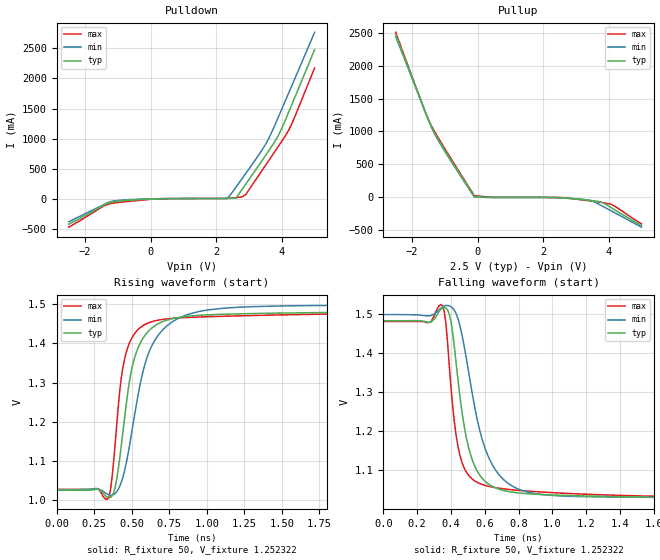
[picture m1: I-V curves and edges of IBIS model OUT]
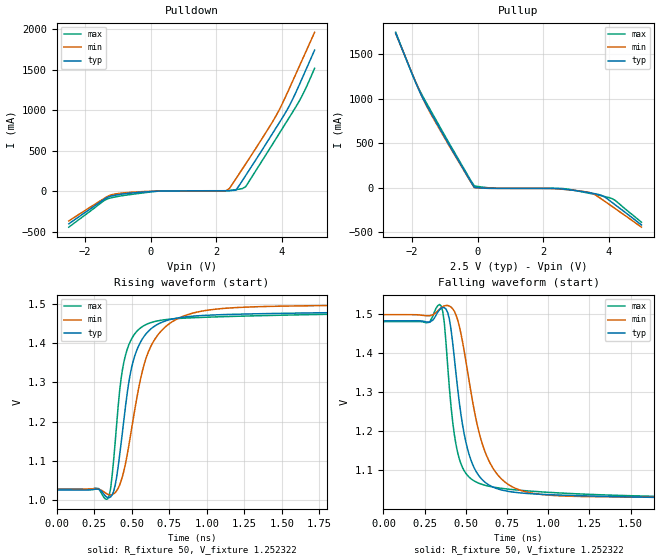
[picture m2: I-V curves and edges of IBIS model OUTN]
|   IBIS File of SG2520VHN D
|   LVDS, Vcc=2.5V, Io=4.5mA, fo<=212.5MHz
[IBIS Ver]   3.2
[File Name]   sg2520vhn_45m_25v.ibs
[File Rev]   1.0
[Date]   Sep. 16, 2020
[Source]
Fairchild Ensigna Lab's Method
[Notes]
Created by Minoru Kozaki
[Disclaimer]
Seiko Epson Corporation makes no warranty with respect to the
information contained herein.
[Copyright]
Copyright(C) 2020, Seiko Epson Corporation. All rights reserved.
|   Component
[Component]   SG2520VHN
[Manufacturer]  Seiko Epson Corporation
[Package]
R_pkg   17.7m   NA   NA
L_pkg   235p   NA   NA
C_pkg   208f   NA   NA
[Pin]   signal_name   model_name   R_pin   L_pin   C_pin
1   OE/ST   NC
2   NC   NC
3   GND   GND
4   OUT   OUT   17.7m   235p   208f
5   OUTN   OUTN   10.4m   129p   221f
6   VCC   POWER
[Diff Pin] inv_pin  vdiff  tdelay_typ
4   5   0   0
| Models and submodels in the file (2): OUT (Output), OUTN (Output)
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|   Model OUT
[Model]   OUT
Model_type   Output
Polarity   Non-Inverting
Vref = 1.25
Vmeas = 1.25
Rref = 50
Cref = 0
C_comp   4.5p   4.5p   4.5p
[Temperature Range]   25   105   -40
[Voltage Range]   2.5   2.25   2.75
[Pullup Reference]   2.5   2.25   2.75
[Pulldown Reference]   0   0   0
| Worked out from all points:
|   slope of the pulldown table from 0 to 0.375 V, typ, clamps not added: 59.1 ohm
|   slope of the pullup table from 0 to 0.375 V, typ, clamps not added: 50.8 ohm
|   falling waveform, R_fixture 50, V_fixture 1.252322: 20-80 % time 108ps typ, 152ps min, 80.6ps max; typ from 1.48 V to 1.03 V
|   rising waveform, R_fixture 50, V_fixture 1.252322: 20-80 % time 122ps typ, 172ps min, 90.6ps max; typ from 1.02 V to 1.48 V
[Pullup]
-2.5V     2.473A     2.445A     2.508A
-1.7V     1.427A     1.43A      1.431A
-1.5V     1.171A     1.177A     1.178A
-1.4V     1.056A     1.057A     1.074A
-1.2V     874.3mA    859.4mA    903.4mA
-100mV    7.183mA    2.067mA    23.14mA
500mV     -4.278mA   -4.465mA   -3.11mA
2.6V      -12.46mA   -13.35mA   -6.641mA
3.4V      -46.9mA    -46.37mA   -56.15mA
3.8V      -81.74mA   -135.1mA   -82.78mA
4.1V      -168.2mA   -215.1mA   -114.4mA
5V        -434.1mA   -456.9mA   -408.4mA
[Pulldown]
-2.5V     -423.2mA   -382mA     -471.3mA
-1.2V     -54.96mA   -42.81mA   -77.17mA
200mV     551.4uA    1.129mA    -537.1uA
2.3V      5.764mA    5.553mA    6.62mA
2.4V      6.809mA    42.1mA     9.291mA
2.6V      12.84mA    192.8mA    19.71mA
2.9V      244.4mA    421.8mA    72mA
3.6V      797.4mA    1.001A     633.7mA
3.9V      1.059A     1.367A     876.2mA
4.1V      1.299A     1.62A      1.04A
4.3V      1.56A      1.874A     1.241A
5V        2.479A     2.767A     2.175A
[Falling Waveform]
R_fixture = 50
V_fixture = 1.252322
V_fixture_min = 1.260634
V_fixture_max = 1.252674
0s        1.483V     1.499V     1.481V
280ps     1.48V      1.497V     1.48V
350ps     1.516V     1.519V     1.522V
370ps     1.516V     1.522V     1.476V
410ps     1.452V     1.516V     1.264V
460ps     1.265V     1.457V     1.127V
540ps     1.111V     1.263V     1.073V
650ps     1.058V     1.11V      1.056V
840ps     1.04V      1.046V     1.047V
4ns       1.026V     1.027V     1.028V
[Rising Waveform]
R_fixture = 50
V_fixture = 1.252322
V_fixture_min = 1.260634
V_fixture_max = 1.252674
0s        1.025V     1.027V     1.028V
340ps     1.007V     1.015V     1.003V
370ps     1.011V     1.013V     1.059V
420ps     1.105V     1.035V     1.275V
460ps     1.231V     1.087V     1.371V
530ps     1.375V     1.24V      1.43V
640ps     1.441V     1.398V     1.456V
800ps     1.465V     1.461V     1.464V
1.1ns     1.474V     1.489V     1.469V
4ns       1.483V     1.499V     1.481V
[Ramp]
R_load = 50
dV/dt_r   0.27069/118.13p   0.27806/164.70p   0.26864/87.59p
dV/dt_f   0.27069/107.33p   0.27806/150.10p   0.26864/79.78p
|   Model OUTN
[Model]   OUTN
Model_type   Output
Polarity   Inverting
Vref = 1.25
Vmeas = 1.25
Rref = 50
Cref = 0
C_comp   4.5p   4.5p   4.5p
[Temperature Range]   25   105   -40
[Voltage Range]   2.5   2.25   2.75
[Pullup Reference]   2.5   2.25   2.75
[Pulldown Reference]   0   0   0
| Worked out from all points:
|   slope of the pulldown table from 0 to 0.375 V, typ, clamps not added: 59.4 ohm
|   slope of the pullup table from 0 to 0.375 V, typ, clamps not added: 51 ohm
|   falling waveform, R_fixture 50, V_fixture 1.252322: 20-80 % time 110ps typ, 153ps min, 82.9ps max; typ from 1.48 V to 1.03 V
|   rising waveform, R_fixture 50, V_fixture 1.252322: 20-80 % time 123ps typ, 172ps min, 91.9ps max; typ from 1.03 V to 1.48 V
[Pullup]
-2.5V     1.739A     1.735A     1.748A
-1.9V     1.192A     1.197A     1.198A
-1.6V     958.4mA    950.8mA    980.2mA
-900mV    504.6mA    494.4mA    522.8mA
-100mV    7.156mA    2.062mA    22.96mA
500mV     -4.278mA   -4.466mA   -3.139mA
2.6V      -12.5mA    -15.04mA   -6.653mA
3.4V      -52.22mA   -49.61mA   -59.2mA
3.6V      -66.09mA   -79.19mA   -73.8mA
3.8V      -85.99mA   -129.7mA   -89.62mA
4.1V      -161.9mA   -206.5mA   -119.2mA
5V        -415.4mA   -440.3mA   -384.8mA
[Pulldown]
-2.5V     -402.6mA   -366.5mA   -443.5mA
-1.4V     -93.83mA   -83.28mA   -109mA
-1.2V     -58.38mA   -44.02mA   -80.47mA
200mV     524.7uA    1.111mA    -583.6uA
2.3V      5.738mA    5.53mA     6.584mA
2.4V      6.77mA     33.85mA    9.231mA
2.6V      12.74mA    155mA      19.53mA
2.9V      195.6mA    338.6mA    57.3mA
3.9V      831mA      987.8mA    698.8mA
4.2V      1.032A     1.242A     892.8mA
4.6V      1.374A     1.601A     1.163A
5V        1.741A     1.961A     1.517A
[Falling Waveform]
R_fixture = 50
V_fixture = 1.252322
V_fixture_min = 1.260634
V_fixture_max = 1.252674
0s        1.483V     1.499V     1.481V
280ps     1.48V      1.496V     1.48V
350ps     1.515V     1.517V     1.522V
390ps     1.504V     1.522V     1.368V
420ps     1.428V     1.514V     1.225V
480ps     1.217V     1.43V      1.107V
550ps     1.107V     1.256V     1.073V
660ps     1.058V     1.109V     1.058V
860ps     1.041V     1.046V     1.048V
4ns       1.026V     1.028V     1.028V
[Rising Waveform]
R_fixture = 50
V_fixture = 1.252322
V_fixture_min = 1.260634
V_fixture_max = 1.252674
0s        1.026V     1.028V     1.028V
340ps     1.007V     1.015V     1.003V
370ps     1.013V     1.014V     1.062V
420ps     1.114V     1.038V     1.278V
460ps     1.241V     1.094V     1.371V
530ps     1.378V     1.25V      1.428V
640ps     1.44V      1.401V     1.454V
820ps     1.465V     1.465V     1.463V
1.15ns    1.473V     1.49V      1.468V
4ns       1.483V     1.499V     1.48V
[Ramp]
R_load = 50
dV/dt_r   0.26900/117.90p   0.27632/163.40p   0.26697/87.97p
dV/dt_f   0.26900/108.41p   0.27632/149.82p   0.26697/81.72p
